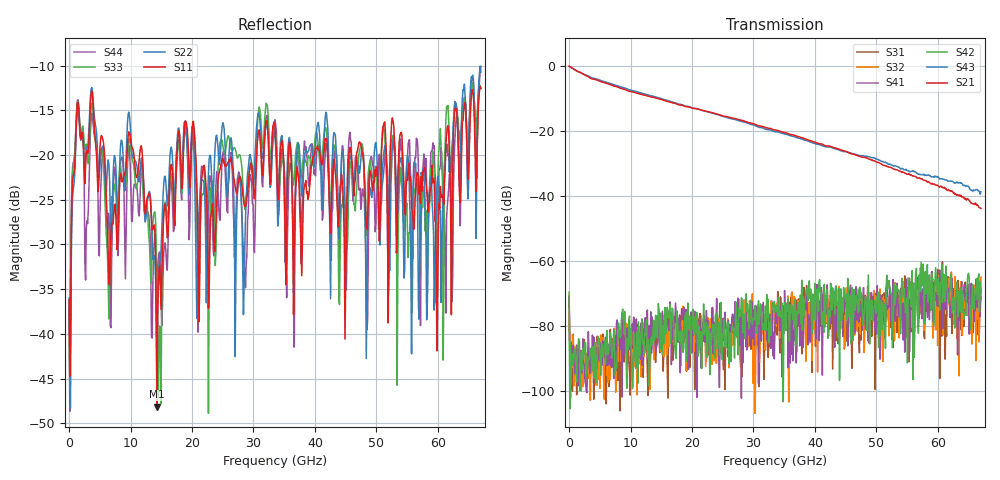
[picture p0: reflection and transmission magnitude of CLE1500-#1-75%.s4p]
!Keysight Technologies,N5247B,US50470101,A.16.20.02
!Date: Thursday, March 13, 2025 10:29:13
!Correction: S11(C  4-Port  )
!S12(C  4-Port  )
!S13(C  4-Port  )
!S14(C  4-Port  )
!S21(C  4-Port  )
!S22(C  4-Port  )
!S23(C  4-Port  )
!S24(C  4-Port  )
!S31(C  4-Port  )
!S32(C  4-Port  )
!S33(C  4-Port  )
!S34(C  4-Port  )
!S41(C  4-Port  )
!S42(C  4-Port  )
!S43(C  4-Port  )
!S44(C  4-Port  )
!S4P File: Measurements: <S11,S12,S13,S14>,
!<S21,S22,S23,S24>,
!<S31,S32,S33,S34>,
!<S41,S42,S43,S44>:
# Hz S  dB  R 50
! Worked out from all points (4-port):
!   601 points, 10 MHz to 67 GHz, reference 50 ohm
!   strongest paths, dB at 10 MHz, 16.76 GHz, 33.51 GHz, 50.25 GHz, 67 GHz:
!     S21: 0.0, -11.3, -19.7, -29.6, -43.8
!     S43: 0.0, -11.0, -20.2, -28.8, -38.7
!     S42: -69.6, -74.5, -73.5, -69.9, -68.9
!     S41: -71.6, -78.8, -78.7, -74.2, -69.0
!     S32: -72.6, -84.9, -79.7, -79.7, -65.0
!     S31: -70.8, -80.7, -78.0, -71.7, -71.2
!   lowest |S11| = -48.2 dB at 14.3 GHz (marker M1), VSWR 1.01, Z = 49.7 - j0.249 ohm
!   |S11| at or under -10 dB: start of sweep to end of sweep
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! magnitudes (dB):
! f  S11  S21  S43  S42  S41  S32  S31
! 10 MHz  -36.2  0.0  0.0  -69.6  -71.6  -72.6  -70.8
! 1.238 GHz  -15.4  -1.5  -1.5  -97.2  -85.9  -88.7  -101.2
! 3.694 GHz  -12.8  -3.9  -3.6  -93.9  -87.7  -88.8  -87.2
! 14.3 GHz  -48.2  -9.9  -9.6  -83.4  -86.1  -77.6  -79.1
! 18.88 GHz  -16.3  -12.4  -12.3  -76.8  -77.4  -82.2  -78.3
! 48.47 GHz  -28.3  -28.3  -27.8  -81.4  -71.7  -74.7  -75.1
! 67 GHz  -12.5  -43.8  -38.7  -68.9  -69.0  -65.0  -71.2
